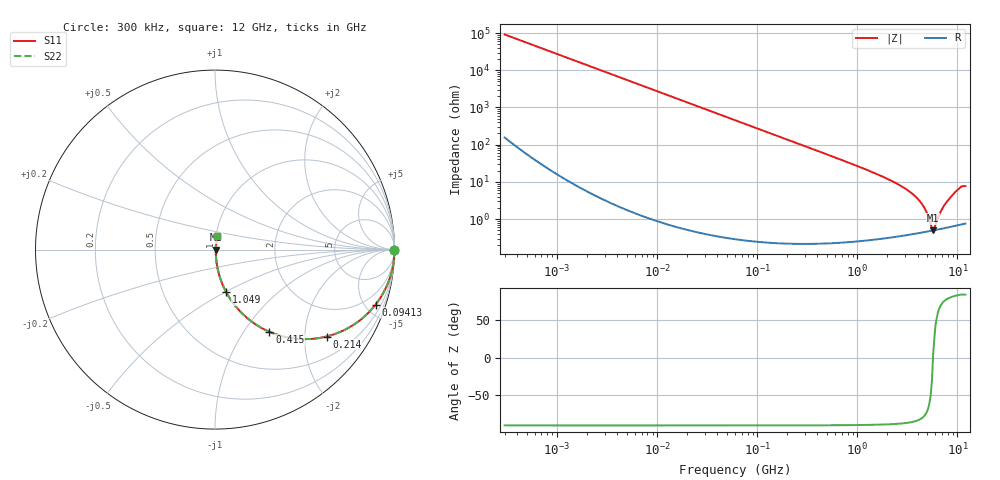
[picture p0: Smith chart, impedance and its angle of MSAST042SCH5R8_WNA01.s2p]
! MSAST042SCH5R8_WNA01  S-PARAMETER MODEL  ( General Type )
! Model Generated by TAIYO YUDEN Corporation (http://www.ty-top.com)
! Version 1.0
! TAIYO YUDEN Control No. 150820
! Copyright(c) 2015 TAIYO YUDEN CO.,LTD. All Rights Reserved.
! Product Description (link to TY-COMPAS)
! https://ds.yuden.co.jp/TYCOMPAS/or/detail?pn=MSAST042SCH5R8BWNA01&u=M
! Products Name : Multilayer Ceramic Capacitors
! Characteristics :
!  Capacitance : 5.8 pF , Rated Voltage : 25V , TCC : CH / C0H
!  Case Size : 0.4 x 0.2 / 0.016 x 0.008 [mm/inch] , Thickness : 0.2 / 0.008 [mm/inch]
!  (Conditions: Temperature = 25 degC , DC Bias Current/Voltage = 0A / 0V)
! External Node Assignments :
!  1  o---| |---o  2
! GND o---------o GND
! Frequency Range : 0.3MHz  -  12000MHz  [ 401 STEP ]
# MHz S RI R 50
! Freq[MHz].  S11 Real  S11 Imag  S21 Real  S21 Imag  S12 Real  S12 Imag  S22 Real  S22 Imag
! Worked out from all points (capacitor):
!   401 points, 300 kHz to 12 GHz, reference 50 ohm
!   read as one part in series: C = 5.8 pF near 316.3 kHz
!   lowest |Z| = 497 mohm at 5.715 GHz (marker M1)
!   series resonance near 5.697 GHz, so ESL is about 130 pH
!   S11 on the Smith chart (normalised r, x): 300 kHz: open; 94.13 MHz: 1.00, -5.83; 214 MHz: 1.00, -2.56; 415 MHz: 1.00, -1.32; 1.049 GHz: 1.01, -0.51; 12 GHz: 1.02, +0.15
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0.3  1 -0.00109  3.05e-06 0.00109  3.05e-06 0.00109  1 -0.00109
1.769972  1 -0.00644  4.43e-05 0.00644  4.43e-05 0.00644  1 -0.00644
10.44266  0.9985 -0.038  0.00146 0.038  0.00146 0.038  0.9985 -0.038
27.82928  0.9898 -0.1003  0.0102 0.1003  0.0102 0.1003  0.9898 -0.1003
60  0.9543 -0.2085  0.0457 0.2085  0.0457 0.2085  0.9543 -0.2085
94.13233  0.8946 -0.3066  0.1054 0.3066  0.1054 0.3066  0.8946 -0.3066
213.9924  0.6213 -0.4842  0.3787 0.4842  0.3787 0.4842  0.6213 -0.4842
353.9943  0.3743 -0.4825  0.6257 0.4825  0.6257 0.4825  0.3743 -0.4825
414.98  0.3029 -0.4579  0.6971 0.4579  0.6971 0.4579  0.3029 -0.4579
651.0506  0.1491 -0.3535  0.8509 0.3535  0.8509 0.3535  0.1491 -0.3535
1048.836  0.0623 -0.2367  0.9377 0.2367  0.9377 0.2367  0.0623 -0.2367
2088.533  0.0158 -0.1118  0.9842 0.1118  0.9842 0.1118  0.0158 -0.1118
3107.553  0.00752 -0.0616  0.9925 0.0616  0.9925 0.0616  0.00752 -0.0616
4050.141  0.00529 -0.0335  0.9947 0.0335  0.9947 0.0335  0.00529 -0.0335
4747.894  0.00481 -0.0179  0.9952 0.0179  0.9952 0.0179  0.00481 -0.0179
5420.343  0.00483 -0.0052  0.9952 0.0052  0.9952 0.0052  0.00483 -0.0052
5715.274  0.00493 0.000369  0.9951 -0.000369  0.9951 -0.000369  0.00493 0.000369
6026.253  0.0051 0.00477  0.9949 -0.00477  0.9949 -0.00477  0.0051 0.00477
6879.757  0.00569 0.0157  0.9943 -0.0157  0.9943 -0.0157  0.00569 0.0157
7854.144  0.00669 0.0287  0.9933 -0.0287  0.9933 -0.0287  0.00669 0.0287
10511.28  0.0115 0.0672  0.9885 -0.0672  0.9885 -0.0672  0.0115 0.0672
12000  0.0132 0.075  0.9868 -0.075  0.9868 -0.075  0.0132 0.075
